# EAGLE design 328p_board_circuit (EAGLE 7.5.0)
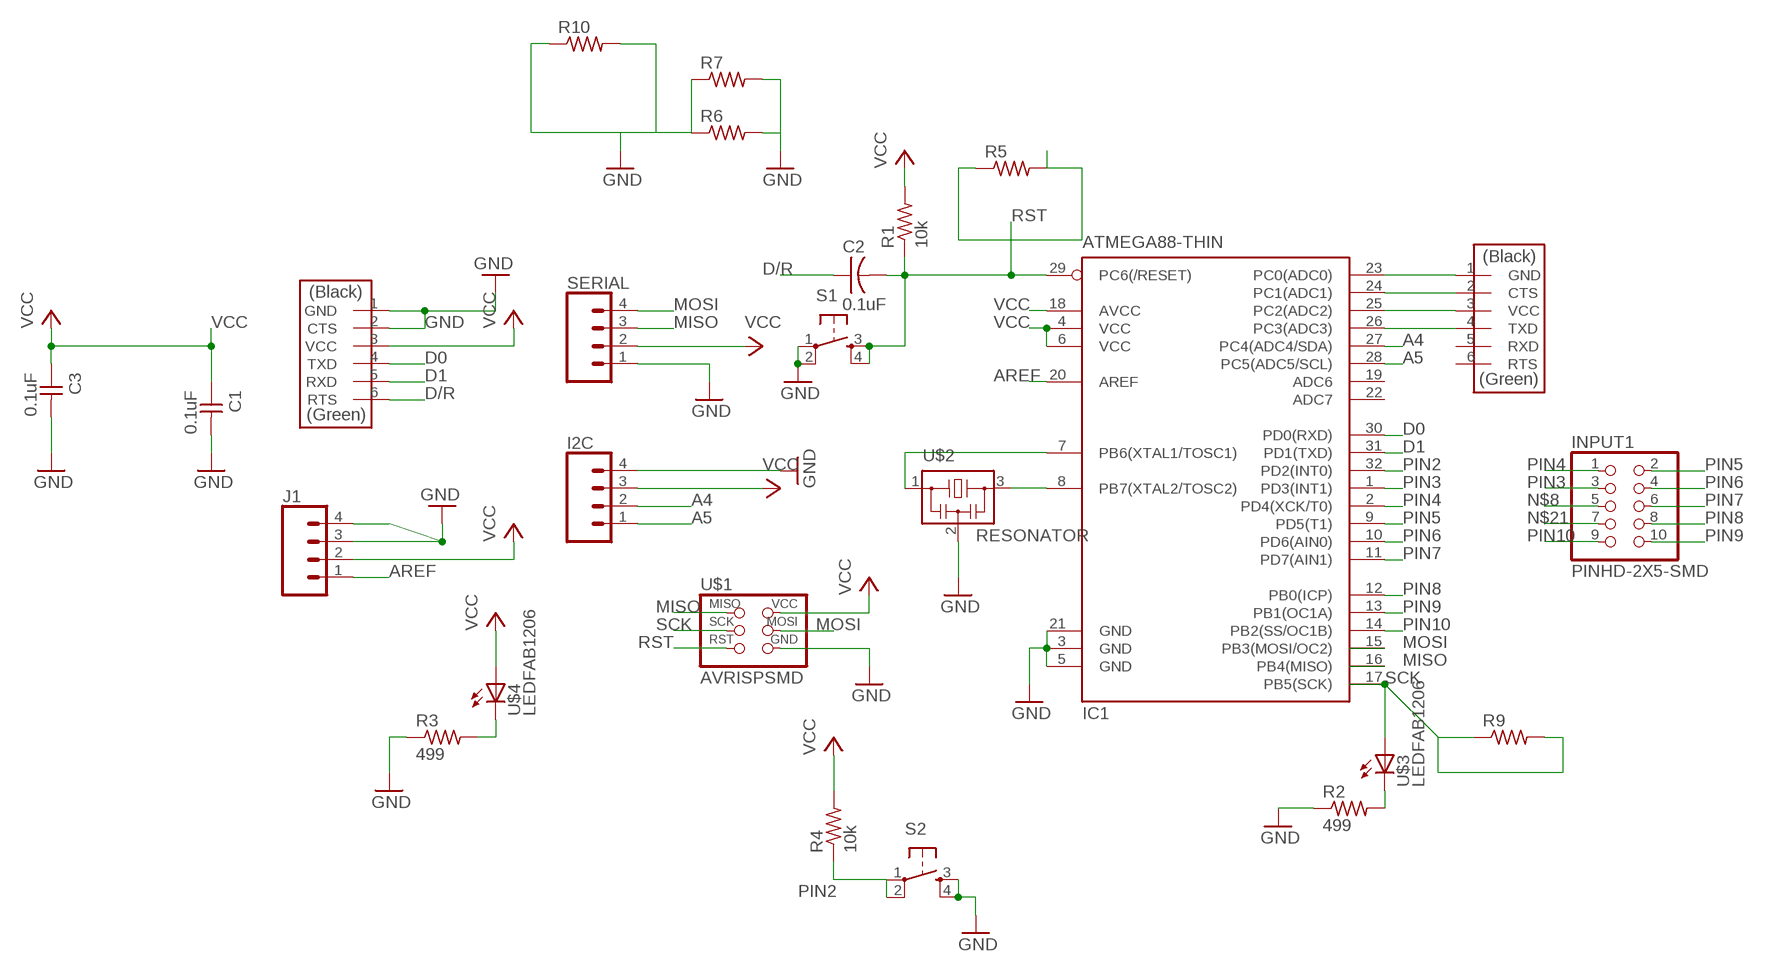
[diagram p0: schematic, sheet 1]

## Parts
C1  0.1uF  CAP-UNPOLARIZEDFAB  [C1206FAB]
C2  0.1uF  CAP-US1206FAB  [C1206FAB]
C3  0.1uF  CAP-UNPOLARIZEDFAB  [C1206FAB]
I2C  CONN_04SMD  [1X04_SMD_RA_MALE]
IC1  ATMEGA88-THIN  [TQFP32-08THIN]
INPUT1  PINHD-2X5-SMD  [2X05SMD]
J1  CONN_04SMD  [1X04_SMD_RA_MALE]
R1  10k  RES-US1206FAB  [R1206FAB]
R2  499  RES-US1206FAB  [R1206FAB]
R3  499  RES-US1206FAB  [R1206FAB]
R4  10k  RES-US1206FAB  [R1206FAB]
R5  RES-US1206FAB  [R1206FAB]
R6  RES-US1206FAB  [R1206FAB]
R7  RES-US1206FAB  [R1206FAB]
R9  RES-US1206FAB  [R1206FAB]
R10  RES-US1206FAB  [R1206FAB]
S1  6MM_SWITCH6MM_SWITCH  [6MM_SWITCH]
S2  6MM_SWITCH6MM_SWITCH  [6MM_SWITCH]
SERIAL  CONN_04SMD  [1X04_SMD_RA_MALE]
U$1  AVRISPSMD  [2X03SMD]
U$2  RESONATOR  [EFOBM]
U$3  LEDFAB1206  [LED1206FAB]
U$4  LEDFAB1206  [LED1206FAB]
U$5  FTDI-SMD-HEADER  [1X06SMD]
U$6  FTDI-SMD-HEADER  [1X06SMD]

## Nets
A4: I2C.2 IC1.27(PC4(ADC4/SDA))
A5: I2C.1 IC1.28(PC5(ADC5/SCL))
AREF: IC1.20(AREF) J1.1
D0: IC1.30(PD0(RXD)) U$6.4(TXD)
D1: IC1.31(PD1(TXD)) U$6.5(RXD)
D/R: C2.1 U$6.6(RTS)
GND: C1.2 C3.2 I2C.4 IC1.3(GND) IC1.5(GND) IC1.21(GND) J1.3 J1.4 R2.1 R3.1 R6.1 R6.2 R7.1 R7.2 R10.1 R10.2 S1.1(P) S1.2(P1) S2.3(S) S2.4(S1) SERIAL.1 U$1.6(GND) U$2.2 U$6.1(GND) U$6.2(CTS)
MISO: IC1.16(PB4(MISO)) SERIAL.3 U$1.1(MISO)
MOSI: IC1.15(PB3(MOSI/OC2)) SERIAL.4 U$1.4(MOSI)
N$1: IC1.23(PC0(ADC0)) U$5.1(GND)
N$2: IC1.24(PC1(ADC1)) U$5.2(CTS)
N$3: IC1.25(PC2(ADC2)) U$5.3(VCC)
N$4: IC1.26(PC3(ADC3)) U$5.4(TXD)
N$8: INPUT1.5
N$11: IC1.8(PB7(XTAL2/TOSC2)) U$2.3
N$12: IC1.7(PB6(XTAL1/TOSC1)) U$2.1
N$13: R2.2 U$3.2(C)
N$14: R3.2 U$4.2(C)
N$21: INPUT1.7
PIN2: IC1.32(PD2(INT0)) R4.1 S2.1(P) S2.2(P1)
PIN3: IC1.1(PD3(INT1)) INPUT1.3
PIN4: IC1.2(PD4(XCK/T0)) INPUT1.1
PIN5: IC1.9(PD5(T1)) INPUT1.2
PIN6: IC1.10(PD6(AIN0)) INPUT1.4
PIN7: IC1.11(PD7(AIN1)) INPUT1.6
PIN8: IC1.12(PB0(ICP)) INPUT1.8
PIN9: IC1.13(PB1(OC1A)) INPUT1.10
PIN10: IC1.14(PB2(SS/OC1B)) INPUT1.9
RST: C2.2 IC1.29(PC6(/RESET)) R1.1 R5.1 R5.2 S1.3(S) S1.4(S1) U$1.5(RST)
SCK: IC1.17(PB5(SCK)) R9.1 R9.2 U$1.3(SCK) U$3.1(A)
VCC: C1.1 C3.1 I2C.3 IC1.4(VCC) IC1.6(VCC) IC1.18(AVCC) J1.2 R1.2 R4.2 SERIAL.2 U$1.2(VCC) U$4.1(A) U$6.3(VCC)
Unconnected: IC1.19(ADC6) IC1.22(ADC7) U$5.5(RXD) U$5.6(RTS)

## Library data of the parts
C1 C3 = fab:CAP-UNPOLARIZED
C2 = fab:CAP-US
I2C J1 SERIAL = SparkFun-Connectors:CONN_04: Multi connection point. Often used as Generic Header-pin footprint for 0.1 inch spaced/style header connections On any of the 0.1 inch spaced packages, you can populate with these: Break Away Headers - Straight (PRT-00116) Break Away Male Headers - Right Angle (PRT-00553) Female Headers (PRT-00115)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; PROD_ID: CONN-09140; SF_ID: PRT-12638
IC1 = fab:ATMEGA88-THIN
INPUT1 = fab:PINHD-2X5-SMD
R1-R7 R9 R10 = fab:RES-US: Resistor (US Symbol)
S1 S2 = fab:6MM_SWITCH: OMRON SWITCH
U$1 = fab:AVRISP
U$2 = fab:RESONATOR
U$3 U$4 = fab:LED: LED
U$5 U$6 = fab:FTDI-SMD-HEADER

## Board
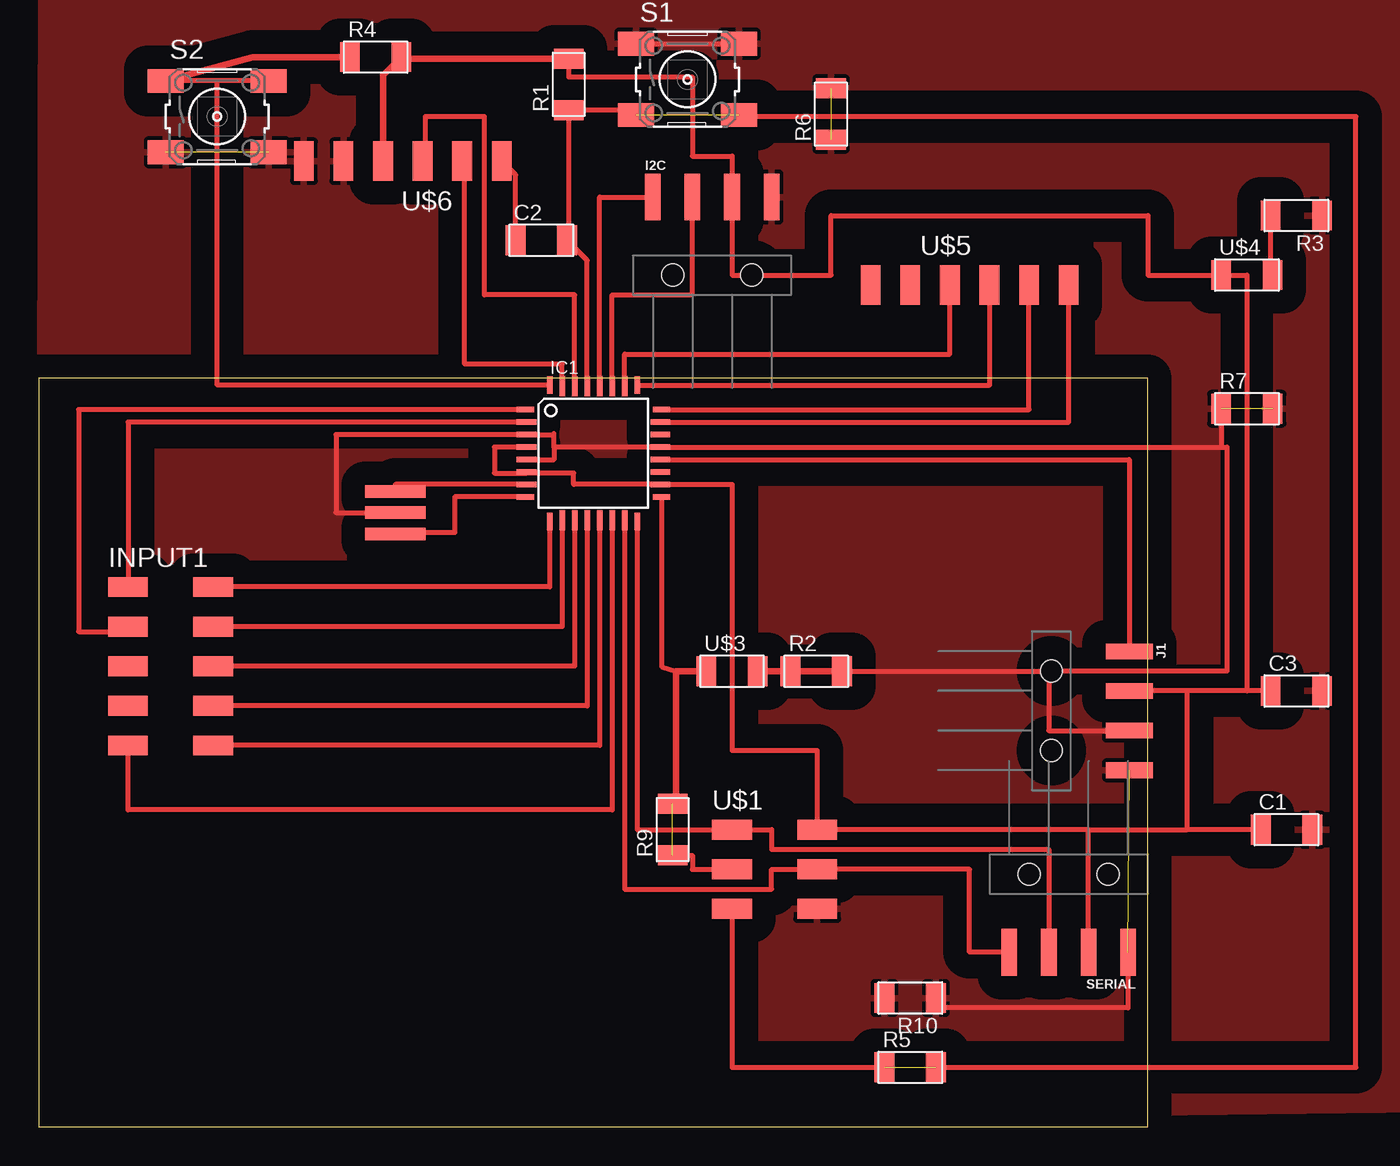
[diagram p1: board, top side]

Size 71.12 x 48.01 mm. Coordinates in mm from the lower left corner, seen from the top.
Outline: 0,0 71.12,0 71.12,48.01 0,48.01 0,0
Copper layers (1*16): Top 0.035mm / dielectric 1.5mm / Bottom 0.035mm
Design rules "default": minimum track width 10mil, minimum drill 24mil, track to track 8mil, track to pad 8mil, pad to pad 8mil, via to via 8mil, smd to smd 8mil, copper to edge 40mil, drill to drill 8mil, minimum pad ring 10mil, minimum via ring 8mil, stop-mask expansion 4mil, vias tented up to drill 0mil, thermal gap 10mil

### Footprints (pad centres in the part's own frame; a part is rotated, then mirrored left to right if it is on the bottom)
C1206FAB = smd 1.27 x 1.905: 1 -1.651,0; 2 1.651,0
1X04_SMD_RA_MALE = smd 1 x 3: 1 -3.81,5; 2 -1.27,5; 3 1.27,5; 4 3.81,5 | hole 1.4: -2.54,0; 2.54,0
TQFP32-08THIN = smd 1.118 x 0.356: 1 -4.369,2.8; 8 -4.369,-2.8; 17 4.369,-2.8; 24 4.369,2.8 | smd 1.27 x 0.356: 2 -4.293,2; 3 -4.293,1.2; 4 -4.293,0.4; 5 -4.293,-0.4; 6 -4.293,-1.2; 7 -4.293,-2; 18 4.293,-2; 19 4.293,-1.2; 20 4.293,-0.4; 21 4.293,0.4; 22 4.293,1.2; 23 4.293,2 | smd 0.356 x 1.118: 9 -2.8,-4.369; 16 2.8,-4.369; 25 2.8,4.369; 32 -2.8,4.369 | smd 0.356 x 1.27: 10 -2,-4.293; 14 1.2,-4.293; 15 2,-4.293; 26 2,4.293; 27 1.2,4.293; 31 -2,4.293 | smd 0.35 x 1.27: 11 -1.2,-4.293; 12 -0.4,-4.293; 13 0.4,-4.293; 28 0.4,4.293; 29 -0.4,4.293; 30 -1.2,4.293
2X05SMD = smd 2.54 x 1.27: 1 -2.54,2.54; 2 2.92,2.54; 3 -2.54,0; 4 2.92,0; 5 -2.54,-2.54; 6 2.92,-2.54; 7 -2.54,-5.08; 8 2.92,-5.08; 9 -2.54,-7.62; 10 2.92,-7.62
R1206FAB = smd 1.27 x 1.905: 1 -1.651,0; 2 1.651,0
6MM_SWITCH = smd 2.286 x 1.524: 1 -3.302,2.286; 2 3.302,2.286; 3 -3.302,-2.286; 4 3.302,-2.286
2X03SMD = smd 2.54 x 1.27: 1 -2.54,2.54; 2 2.92,2.54; 3 -2.54,0; 4 2.92,0; 5 -2.54,-2.54; 6 2.92,-2.54
EFOBM = smd 0.8 x 3.9: 1 -1.35,0; 2 0,0; 3 1.35,0
LED1206FAB = smd 1.27 x 1.905: 1 -1.651,0; 2 1.651,0
1X06SMD = smd 2.54 x 1.27: 1 0,6.35; 2 0,3.81; 3 0,1.27; 4 0,-1.27; 5 0,-3.81; 6 0,-6.35

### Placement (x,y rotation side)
C1  80.01,19.05 0 top  (outside the outline)
C2  32.23,56.83 0 top  (outside the outline)
C3  80.64,27.94 0 top  (outside the outline)
I2C  43.18,54.61 0 top  (outside the outline)
IC1  35.56,43.18 0 top
INPUT1  8.26,32.07 0 top
J1  64.93,26.67 270 top
R1  33.97,66.83 90 top  (outside the outline)
R2  49.85,29.21 0 top
R3  80.64,58.42 180 top  (outside the outline)
R4  21.59,68.58 0 top  (outside the outline)
R5  55.88,3.81 0 top
R6  not placed on the board
R7  77.47,46.04 0 top  (outside the outline)
R9  40.64,19.05 90 top
R10  55.88,8.26 180 top
S1  41.59,67.15 0 top  (outside the outline)
S2  11.43,64.77 0 top  (outside the outline)
SERIAL  66.04,16.19 180 top
U$1  46.99,16.51 0 top
U$2  22.86,39.37 270 top
U$3  44.45,29.21 0 top
U$4  77.47,54.61 0 top  (outside the outline)
U$5  59.69,53.98 270 top  (outside the outline)
U$6  23.34,61.91 90 top  (outside the outline)

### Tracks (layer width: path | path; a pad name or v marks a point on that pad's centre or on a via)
A4
  Top 0.305: IC1.27 36.76,53.34 41.91,53.34 I2C.2
A5
  Top 0.305: IC1.28 35.96,59.61 I2C.1
AREF
  Top 0.305: IC1.20 69.93,42.78 J1.1
D0
  Top 0.305: IC1.30 34.36,53.34 28.57,53.34 28.57,64.77 24.77,64.77 24.77,61.91 U$6.4
D1
  Top 0.305: IC1.31 33.56,48.9 27.3,48.9 27.3,61.91 U$6.5
D/R
  Top 0.305: C2.1 30.57,61.02 U$6.6
GND  (4 unrouted)
  Top 0.305: U$2.2 19.05,39.37 19.05,44.38 IC1.3 33.02,44.38 | S1.1 S1.2 | IC1.5 33.02,42.78 33.02,43.58 | 33.02,43.58 33.02,44.38 | 33.02,44.38 33.02,44.45 | 33.02,43.58 IC1.21 75.82,43.58 | 64.77,29.21 76.2,29.21 76.2,43.58 75.82,43.58 | 64.77,29.21 64.77,25.4 J1.3 | R2.1 64.77,29.21 | SERIAL.1 69.85,7.62 57.53,7.62 R10.1 | R7.1 75.82,43.58
  pour Top (isolate 1.524): 0,0 88.9,1.11 89.06,75.56 0.16,75.72
MISO
  Top 0.305: IC1.16 38.36,19.05 U$1.1 46.99,19.05 46.99,17.78 64.77,17.78 SERIAL.3
MOSI
  Top 0.305: SERIAL.4 59.69,11.19 59.69,16.51 U$1.4 46.99,16.51 46.99,15.24 37.56,15.24 IC1.15
N$1
  Top 0.305: IC1.23 66.04,45.18 U$5.1
N$2
  Top 0.305: IC1.24 63.5,45.98 U$5.2
N$3
  Top 0.305: U$5.3 60.96,47.55 IC1.25
N$4
  Top 0.305: IC1.26 37.56,49.53 58.42,49.53 U$5.4
N$11
  Top 0.305: IC1.8 26.67,40.38 26.67,38.1 22.86,38.1 U$2.3
N$12
  Top 0.305: IC1.7 22.86,41.18 U$2.1
N$13
  Top 0.406: U$3.2 R2.2
N$14
  Top 0.305: U$4.2 78.99,54.61 R3.2
PIN2
  Top 0.305: S2.2 11.43,67.06 | 11.43,67.06 S2.1 | 11.43,67.06 11.43,47.55 IC1.32
  Top 0.406: R4.1 13.72,68.58 S2.1
PIN3
  Top 0.305: IC1.1 2.54,45.98 2.54,31.75 5.71,31.75 INPUT1.3
PIN4
  Top 0.305: IC1.2 5.71,45.18 INPUT1.1
PIN5
  Top 0.305: IC1.9 32.76,34.61 INPUT1.2
PIN6
  Top 0.305: IC1.10 33.56,32.07 INPUT1.4
PIN7
  Top 0.305: IC1.11 34.36,29.53 INPUT1.6
PIN8
  Top 0.305: IC1.12 35.16,26.99 INPUT1.8
PIN9
  Top 0.305: IC1.13 35.96,24.45 INPUT1.10
PIN10
  Top 0.305: IC1.14 36.76,20.32 5.71,20.32 INPUT1.9
RST  (2 unrouted)
  Top 0.305: S1.3 38.29,65.18 R1.1 33.97,56.83 C2.2 35.16,55.55 IC1.29 | U$1.5 44.45,3.81 R5.1 | R5.2 84.45,3.81 84.45,64.77 44.9,64.77 S1.4
SCK  (1 unrouted)
  Top 0.305: IC1.17 39.93,29.51 40.86,29.21 | R9.1 41.91,17.4 41.91,16.51 U$1.3
  Top 0.406: U$3.1 40.86,29.21 40.86,20.92 R9.2
VCC
  Top 0.305: IC1.4 29.21,43.58 29.21,41.91 31.27,41.91 | 31.27,41.91 34.29,41.91 34.29,41.18 IC1.18 44.45,41.18 44.45,24.13 49.91,24.13 U$1.2 67.31,19.05 | 31.27,41.91 IC1.6 | 77.47,27.94 77.47,54.61 U$4.1 71.12,54.61 71.12,58.42 50.8,58.42 50.8,54.61 44.45,54.61 I2C.3 44.45,62.23 41.91,62.23 41.91,67.31 33.97,67.31 R1.2 | 73.66,27.94 J1.2 | SERIAL.2 67.31,19.05 | 67.31,19.05 73.66,19.05 | 73.66,19.05 73.66,27.94 | C1.1 73.66,19.05 | 77.47,27.94 73.66,27.94 | C3.1 77.47,27.94
  Top 0.406: U$6.3 22.07,67.41 R4.2 23.24,68.48 R1.2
